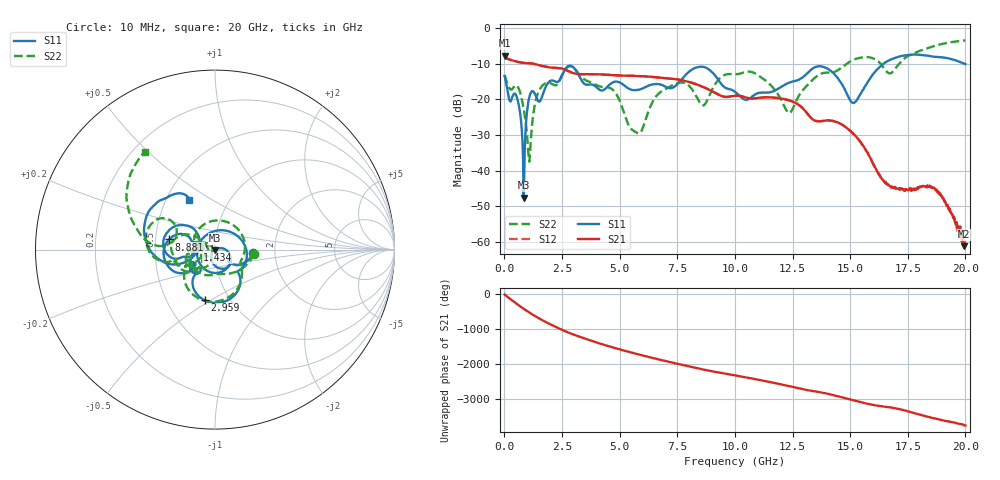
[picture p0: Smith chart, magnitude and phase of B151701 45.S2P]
!  2-Port S-parameters saved by WinCal
! VAR MeasName=S-Parameters (CALIBRATED_DATA) read from VNA (N5244A)
! VAR MeasDate=2015-12-24 19:14:45
! VAR NAME=B151701 45
! VAR FILENAME=B151701 45.S2P
! VAR DATE=2015-12-24 19:14:45
! VAR PHYS_PORTS=1,3
# Hz S DB R 50
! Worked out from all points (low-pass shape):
!   801 points, 10 MHz to 20 GHz, reference 50 ohm
!   highest |S21| = -7.78 dB at 10 MHz (marker M1); lowest = -61.2 dB at 19.93 GHz (marker M2)
!   |S21| within 3 dB of the highest: start of sweep to 1.751 GHz
!   lowest |S11| = -47.5 dB at 834.6 MHz (marker M3), VSWR 1.01, Z = 49.8 - j0.362 ohm
!   |S11| at or under -10 dB: start of sweep to 16.45 GHz; 19.97341 GHz to end of sweep
!   |S22| runs from -37.5 to -3.5 dB; largest |S21 - S12| = 0.0014
!   S11 on the Smith chart (normalised r, x): 10 MHz: 1.54, -0.06; 1.434 GHz: 0.82, -0.00; 2.959 GHz: 0.76, -0.47; 8.881 GHz: 0.59, +0.07; 20 GHz: 0.65, +0.40
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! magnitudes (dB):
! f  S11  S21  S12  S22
! 10 MHz  -13.4  -7.8  -7.8  -13.2
! 559.7 MHz  -19.8  -9.5  -9.5  -16.3
! 834.6 MHz  -47.5  -9.8  -9.8  -22.6
! 1.084 GHz  -19.3  -9.9  -9.9  -37.5
! 1.434 GHz  -20.1  -10.3  -10.3  -18.6
! 2.959 GHz  -10.8  -12.6  -12.6  -11.0
! 3.358 GHz  -14.8  -12.9  -12.9  -13.8
! 4.733 GHz  -15.2  -13.2  -13.2  -17.5
! 5.782 GHz  -17.3  -13.4  -13.4  -29.5
! 6.682 GHz  -15.7  -13.9  -13.9  -18.4
! 7.706 GHz  -14.3  -14.6  -14.7  -15.3
! 8.881 GHz  -11.6  -17.3  -17.3  -19.1
! 10.01 GHz  -17.9  -19.0  -19.0  -13.0
! 11.13 GHz  -18.1  -19.5  -19.5  -13.8
! 12.35 GHz  -15.3  -20.3  -20.3  -23.8
! 13.35 GHz  -11.4  -25.5  -25.5  -14.6
! 14.18 GHz  -12.1  -26.0  -26.0  -12.5
! 15.15 GHz  -21.0  -29.7  -29.7  -8.9
! 16.68 GHz  -9.1  -44.0  -44.0  -12.7
! 18.65 GHz  -8.0  -44.8  -45.1  -5.0
! 19.93 GHz  -9.9  -61.2  -59.3  -3.5
! 20 GHz  -10.1  -60.4  -60.9  -3.5
